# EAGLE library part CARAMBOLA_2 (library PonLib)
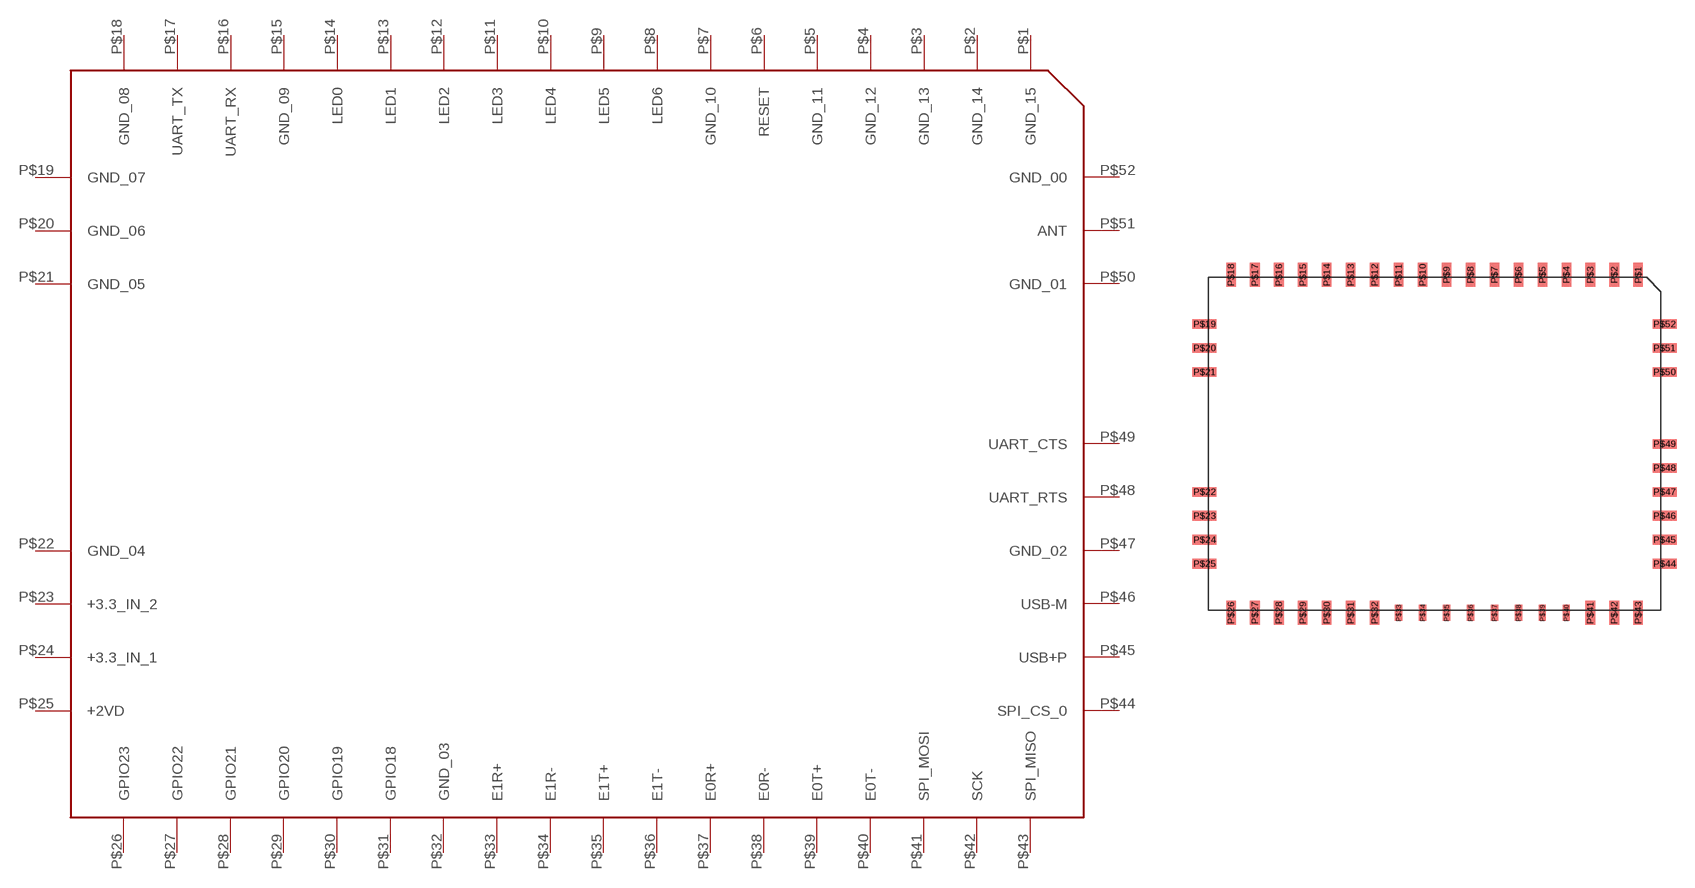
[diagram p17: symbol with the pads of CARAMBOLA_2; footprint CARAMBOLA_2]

Designator prefix -

## CARAMBOLA_2  [CARAMBOLA_2]
P$1  GND_15
P$2  GND_14
P$3  GND_13
P$4  GND_12
P$5  GND_11
P$6  RESET
P$7  GND_10
P$8  LED6
P$9  LED5
P$10  LED4
P$11  LED3
P$12  LED2
P$13  LED1
P$14  LED0
P$15  GND_09
P$16  UART_RX
P$17  UART_TX
P$18  GND_08
P$19  GND_07
P$20  GND_06
P$21  GND_05
P$22  GND_04
P$23  +3.3_IN_2
P$24  +3.3_IN_1
P$25  +2VD
P$26  GPIO23
P$27  GPIO22
P$28  GPIO21
P$29  GPIO20
P$30  GPIO19
P$31  GPIO18
P$32  GND_03
P$33  E1R+
P$34  E1R-
P$35  E1T+
P$36  E1T-
P$37  E0R+
P$38  E0R-
P$39  E0T+
P$40  E0T-
P$41  SPI_MOSI
P$42  SCK
P$43  SPI_MISO
P$44  SPI_CS_0
P$45  USB+P
P$46  USB-M
P$47  GND_02
P$48  UART_RTS
P$49  UART_CTS
P$50  GND_01
P$51  ANT
P$52  GND_00

## Footprint CARAMBOLA_2 (pad centres in mm)
smd 0.8 x 2: P$1 17,14.1; P$2 15,14.1; P$3 13,14.1; P$4 11,14.1; P$5 9,14.1; P$6 7,14.1; P$7 5,14.1; P$8 3,14.1; P$9 1,14.1; P$10 -1,14.1; P$11 -3,14.1; P$12 -5,14.1; P$13 -7,14.1; P$14 -9,14.1; P$15 -11,14.1; P$16 -13,14.1; P$17 -15,14.1; P$18 -17,14.1; P$26 -17,-14.1; P$27 -15,-14.1; P$28 -13,-14.1; P$29 -11,-14.1; P$30 -9,-14.1; P$31 -7,-14.1; P$32 -5,-14.1; P$41 13,-14.1; P$42 15,-14.1; P$43 17,-14.1
smd 2 x 0.8: P$19 -19.2,10; P$20 -19.2,8; P$21 -19.2,6; P$22 -19.2,-4; P$23 -19.2,-6; P$24 -19.2,-8; P$25 -19.2,-10; P$44 19.2,-10; P$45 19.2,-8; P$46 19.2,-6; P$47 19.2,-4; P$48 19.2,-2; P$49 19.2,0; P$50 19.2,6; P$51 19.2,8; P$52 19.2,10
smd 0.61 x 1.321: P$33 -3,-14.1; P$34 -1,-14.1; P$35 1,-14.1; P$36 3,-14.1; P$37 5,-14.1; P$38 7,-14.1; P$39 9,-14.1; P$40 11,-14.1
